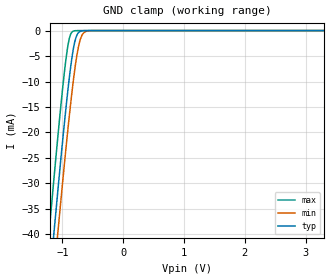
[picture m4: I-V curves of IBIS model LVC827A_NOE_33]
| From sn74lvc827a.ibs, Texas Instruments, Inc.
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[Model]   LVC827A_NOE_33
Model_type  Input
Vinl = 0.8
Vinh = 2
| variable   typ   min   max
C_comp   3.88pF   3.04pF   4.73pF
[Temperature Range]   40   100   -40
| Ambient temperature   25   85   -40
[Voltage range]   3.3   3   3.6
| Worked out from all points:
|   GND clamp passes 1 mA (typ) near -0.77 V on its own axis
[GND Clamp]
| LVC827A_NOE_33
|   Voltage   I(typ)   I(min)   I(max)
-5V       -584.4mA   -591.4mA   -575.6mA
-1.215V   -49.64mA   -57.94mA   -39mA
-1.14V    -39.76mA   -48.06mA   -29.1mA
-1.08V    -32.01mA   -40.28mA   -21.4mA
-1.06V    -29.47mA   -37.73mA   -18.9mA
-925mV    -13.31mA   -21.13mA   -4.126mA
-875mV    -8.132mA   -15.46mA   -1.066mA
-820mV    -3.582mA   -9.784mA   -109.5uA
-770mV    -1.129mA   -5.45mA    -10.74uA
-715mV    -205.6uA   -2.13mA    -809.3nA
-590mV    -2.703uA   -81.94uA   -2.258nA
3.3V      11.73pA    9.26pA     5.93pA
